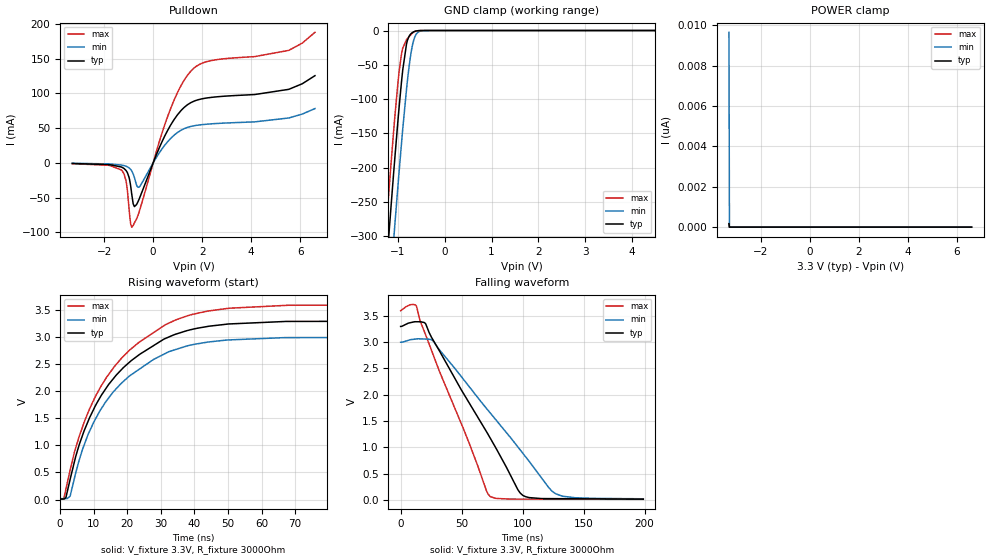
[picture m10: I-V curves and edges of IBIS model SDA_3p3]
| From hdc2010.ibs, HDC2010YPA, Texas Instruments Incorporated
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[Model]   SDA_3p3
Model_type   I/O_open_drain
Polarity   Non-Inverting
Enable   Active-Low
Vinl = .99
Vinh = 2.31
Vmeas = 1.65
Vref = 3.3
Cref = 15pF
Rref = 3000
|   typ   min   max
|   (nom PVT)   (slow PVT)   (fast PVT)
C_comp   1.615p   1.567p   1.665p
|C_comp (ON state)   1.615p   1.567p   1.665p
|C_comp (OFF state)   1.860p   1.794p   1.898p
[Model spec]
|subparameter
Vinl   0.99   0.90   1.08
Vinh   2.31   2.10   2.52
[Voltage Range]   3.3   3   3.6
[Temperature Range]   27   125   -40
[Pullup Reference]   3.3   3   3.6
[Pulldown Reference]   0   -0   -0
[Power Clamp Reference]   3.3   3   3.6
[GND Clamp Reference]   0   0   0
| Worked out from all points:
|   slope of the pulldown table from 0 to 0.495 V, typ, clamps not added: 12.3 ohm
|   GND clamp passes 1 mA (typ) near -0.63 V on its own axis
|   falling waveform, V_fixture 3.3V, R_fixture 3000Ohm: 20-80 % time 49.1ns typ, 61.4ns min, 37.2ns max; typ from 3.3 V to 0.011 V
|   rising waveform, V_fixture 3.3V, R_fixture 3000Ohm: 20-80 % time 18.7ns typ, 18.4ns min, 19.4ns max; typ from 0.009 V to 3.3 V
[Pulldown]
|   Voltage   I(typ)   I(min)   I(max)
-3.3V     -907.1uA   -589.2uA   -1.176mA
-1.29V    -6.095mA   -3.196mA   -10.54mA
-1.102V   -11.28mA   -4.957mA   -27.16mA
-924mV    -31.83mA   -9.258mA   -86.46mA
-874.5mV  -45.07mA   -11.68mA   -92.67mA
-765.6mV  -63.05mA   -21.31mA   -86.47mA
-577.5mV  -52.62mA   -34.96mA   -71.3mA
580.8mV   46.16mA    30.05mA    65.88mA
1.541V    86.88mA    52.53mA    132.4mA
2.373V    94.37mA    56.24mA    147.4mA
5.521V    105.9mA    64.62mA    162mA
6.6V      125.6mA    78.2mA     188.1mA
[GND Clamp]
|   Voltage   I(typ)   I(min)   I(max)
-3.3V     -2.342A    -2.43A     -2.286A
-1.261V   -360.8mA   -459.5mA   -297.6mA
-1.231V   -333.6mA   -432.4mA   -270.4mA
-1.142V   -253.4mA   -351.9mA   -191mA
-1.073V   -193.1mA   -290.7mA   -132.5mA
-993.3mV  -127.7mA   -222.8mA   -72.94mA
-924mV    -76.16mA   -166.1mA   -35.1mA
-815.1mV  -19.72mA   -85.94mA   -13.4mA
-735.9mV  -5.94mA    -40.48mA   -7.156mA
-656.7mV  -1.741mA   -13.1mA    -2.166mA
-399.3mV  -2.817uA   -63.31uA   -438.2nA
6.6V      0A         0A         0A
[POWER Clamp]
|   Voltage   I(typ)   I(min)   I(max)
-3.3V     173.2pA    9.65nA     140.3pA
-3.28V    0A         0A         0A
-3.27V    0A         0A         0A
6.6V      0A         0A         0A
[Ramp]
R_load = 3000
|   typ   min   max
dV/dt_r   1.97439/1.87078e-08   1.79094/1.81291e-08   2.15784/1.94283e-08
dV/dt_f   1.97304/4.90956e-08   1.78884/6.13981e-08   2.1546/3.72721e-08
[Falling Waveform]
V_fixture = 3.3V
V_fixture_min = 3V
V_fixture_max = 3.6V
R_fixture = 3000Ohm
C_fixture = 0F
|   Time   V(typ)   V(min)   V(max)
0s        3.3V       3V         3.599V
12.88ns   3.39V      3.061V     3.691V
20.28ns   3.358V     3.06V      3.154V
26.3ns    3.055V     3.031V     2.785V
73.49ns   1.174V     1.653V     62.13mV
96.4ns    182.4mV    998.6mV    13.03mV
102.6ns   57.36mV    814.3mV    12.74mV
124ns     21.43mV    168.4mV    11.74mV
132.8ns   20.26mV    67.42mV    11.33mV
199ns     11.5mV     18.59mV    8.235mV
[Rising Waveform]
V_fixture = 3.3V
V_fixture_min = 3V
V_fixture_max = 3.6V
R_fixture = 3000Ohm
C_fixture = 0F
|   Time   V(typ)   V(min)   V(max)
0s        9.348mV    15.07mV    3.606mV
1.139ns   10.61mV    17.17mV    31.63mV
2.914ns   357.1mV    58.73mV    528.9mV
5.698ns   1.015V     732.3mV    1.17V
8.225ns   1.43V      1.185V     1.593V
13.81ns   2.066V     1.823V     2.254V
23.36ns   2.665V     2.396V     2.895V
38.16ns   3.124V     2.841V     3.396V
67.95ns   3.287V     2.989V     3.586V
199ns     3.3V       3V         3.6V
